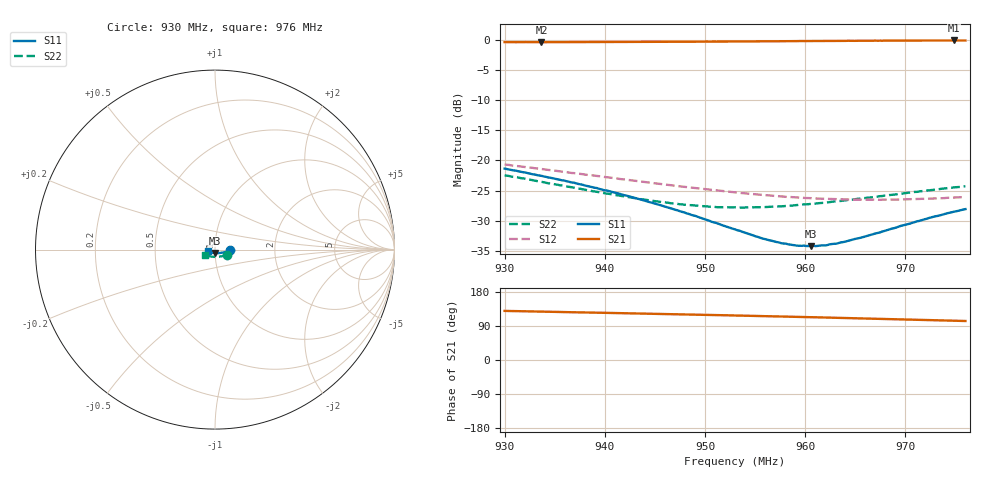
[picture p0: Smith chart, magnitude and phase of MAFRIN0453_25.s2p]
!Part Number:  MAFRIN0453
!Name:  MariaCraven
!Comments:  1
!Thu 30/Sep/2004 11:27:39 AM
!Temperature:  25
# MHZ  S  DB  R  50
!Freq  S11(dB)  S11(ang)  S21(dB)  S21(ang)  S12(dB)  S12(ang)  S22(dB)  S22(ang)
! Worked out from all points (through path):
!   201 points, 930 MHz to 976 MHz, reference 50 ohm
!   highest |S21| = -0.02 dB at 974.85 MHz (marker M1); lowest = -0.3 dB at 933.68 MHz (marker M2)
!   lowest |S11| = -34.3 dB at 960.59 MHz (marker M3), VSWR 1.04, Z = 49.7 - j1.91 ohm
!   |S11| at or under -10 dB: start of sweep to end of sweep
!   |S22| runs from -27.8 to -22.5 dB; largest |S21 - S12| = 0.97
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930  -21.35 -3.3  -0.30 129.6  -20.65 108.0  -22.48 -22.5
933.68  -22.56 -6.8  -0.31 127.7  -21.42 108.7  -23.55 -29.2
937.82  -24.06 -11.6  -0.30 125.5  -22.29 110.5  -24.81 -38.3
941.5  -25.55 -16.7  -0.28 123.6  -23.08 112.4  -25.86 -48.0
945.41  -27.38 -23.7  -0.26 121.6  -23.88 115.7  -26.86 -60.1
949.55  -29.54 -34.4  -0.23 119.4  -24.70 119.8  -27.60 -74.5
951.16  -30.42 -39.8  -0.21 118.5  -24.99 121.7  -27.77 -80.8
953  -31.46 -47.3  -0.19 117.5  -25.31 124.1  -27.79 -87.8
955.76  -33.00 -62.0  -0.17 115.9  -25.73 128.0  -27.77 -98.2
957.6  -33.77 -73.9  -0.15 114.8  -25.99 130.9  -27.64 -104.9
959.21  -34.18 -85.9  -0.13 113.8  -26.17 133.5  -27.41 -110.5
960.59  -34.26 -96.6  -0.12 113.1  -26.27 135.8  -27.22 -115.2
960.82  -34.19 -98.5  -0.12 112.9  -26.30 136.1  -27.20 -115.9
961.05  -34.26 -99.8  -0.12 112.7  -26.32 136.5  -27.18 -116.6
961.97  -34.14 -106.8  -0.11 112.1  -26.39 138.0  -27.04 -119.6
962.43  -33.96 -110.3  -0.10 111.9  -26.41 138.8  -26.92 -120.9
963.12  -33.85 -115.0  -0.09 111.5  -26.44 140.0  -26.80 -123.0
965.65  -32.81 -130.5  -0.07 109.9  -26.54 144.3  -26.32 -129.9
968.41  -31.48 -143.3  -0.06 108.1  -26.53 148.7  -25.76 -137.2
971.17  -30.11 -153.2  -0.04 106.2  -26.43 153.0  -25.23 -143.1
974.85  -28.54 -162.9  -0.02 103.7  -26.17 158.2  -24.49 -150.5
976  -28.10 -165.5  -0.03 102.9  -26.09 159.6  -24.30 -152.4
